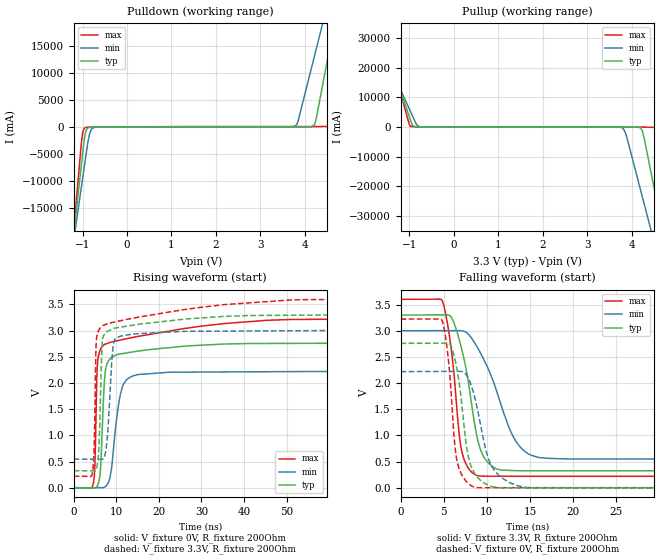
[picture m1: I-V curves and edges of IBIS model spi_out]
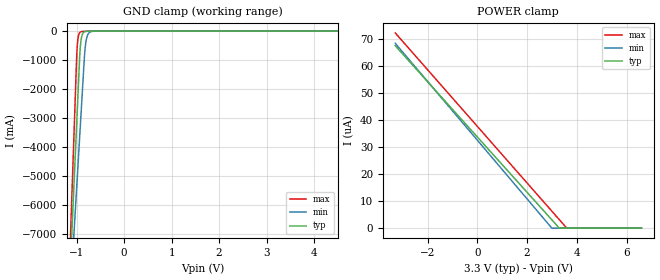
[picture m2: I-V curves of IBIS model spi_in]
|Texas Instruments Incorporated
| Part Name   Digital Voltage Range   Package-type   #pins
| DRV3245AQPHPRQ1   3 - 3.6 V   HTQFP   48
[IBIS Ver]   4.1
[File name]   drv3245_q1.ibs
[File Rev]   1.0
[Date]   06/05/2019
[Source]
| Texas Instruments Incorporated.
| 12500 TI Blvd
| Dallas, TX -75243
[Notes]   Revision History:
| Rev 1.0: 06/05/2019
| - Initial version of the model
| - Model generated from simulations in TISPICE/SPECTRE
| - C_comp although listed in numerical order of value are
|   obtained from varying PVT conditions. For PVT conditions for
|   each specific value refer the buffer description under
|   respective [Model]. IBIS model user is responsible for using
|   appropriate C_comp to simulate for Signal Integrity.
| - Warnings regarding combined Non-monotonicity of various models have been
|   reviewed and considered minor and can be ignored.
[Disclaimer]
| This model is designed as an aid for customers of Texas Instruments.
| TI and its licensors and suppliers make no warranties, either expressed
| or implied, with respect to this  model, including the warranties of
| merchantability or fitness for a particular purpose. The model is
| provided solely on an "as is" basis. The entire risk as to its quality
| and performance is with the customer.
| This model is subject to change without notice. Texas Instruments
| Incorporated is not responsible for updating this model.
[Copyright]
 (C) Copyright 2019 Texas Instruments Incorporated. All rights reserved.
|   DRV3245QPHPRQ1
[Component] DRV3245QPHPRQ1
[Manufacturer]   TI
[Package]
| variable   typ   min   max
R_pkg   0.05   0.04   0.06
L_pkg   1.0nH   0.8nH   1.2nH
C_pkg   0.2pF   0.16pF   0.24pF
| pin number (pin name) mapping to model name
[Pin]   signal_name   model_name   R_pin   L_pin   C_pin
1   EN   NC   NA   NA   NA
2   INHA   NC   NA   NA   NA
3   INLA   NC   NA   NA   NA
4   INHB   NC   NA   NA   NA
5   INLB   NC   NA   NA   NA
6   INHC   NC   NA   NA   NA
7   INLC   NC   NA   NA   NA
8   nFAULT   NC   NA   NA   NA
9   nSCS   spi_in   NA   NA   NA
10   SDI   spi_in   NA   NA   NA
11   SDO   spi_out   NA   NA   NA
12   SCLK   spi_in   NA   NA   NA
13   VDDIO   NC   NA   NA   NA
14   GND   GND   NA   NA   NA
15   AVDD   POWER   NA   NA   NA
16   SO1   NC   NA   NA   NA
17   SO2   NC   NA   NA   NA
18   SO3   NC   NA   NA   NA
19   SN3   NC   NA   NA   NA
20   SP3   NC   NA   NA   NA
21   SN2   NC   NA   NA   NA
22   SP2   NC   NA   NA   NA
23   SN1   NC   NA   NA   NA
24   SP1   NC   NA   NA   NA
25   GLC   NC   NA   NA   NA
26   SLC   NC   NA   NA   NA
27   SHC   NC   NA   NA   NA
28   GHC   NC   NA   NA   NA
29   GHB   NC   NA   NA   NA
30   SHB   NC   NA   NA   NA
31   SLB   NC   NA   NA   NA
32   GLB   NC   NA   NA   NA
33   GLA   NC   NA   NA   NA
34   SLA   NC   NA   NA   NA
35   SHA   NC   NA   NA   NA
36   GHA   NC   NA   NA   NA
37   VCP_LSD   NC   NA   NA   NA
38   VCPH   NC   NA   NA   NA
39   CP2H   NC   NA   NA   NA
40   CP2L   NC   NA   NA   NA
41   PVDD   NC   NA   NA   NA
42   CP1L   NC   NA   NA   NA
43   CP1H   NC   NA   NA   NA
44   VDRAIN   NC   NA   NA   NA
45   GND   NC   NA   NA   NA
46   DVDD   NC   NA   NA   NA
47   DRVOFF   NC   NA   NA   NA
48   VREF   NC   NA   NA   NA
| Models and submodels in the file (2): spi_out (Output), spi_in (Input)
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|   Model
[Model]   spi_out
Model_type   Output
Polarity   Non-Inverting
Vmeas = 1.65
Vref = 1.65
Cref = 15pF
Rref = 1000000
|   typ   min   max
C_comp   2.7pF   2.5pF   2.9pF
[Voltage Range]   3.3   3   3.6
[Temperature Range]   27   125   -40
[Pullup Reference]   3.3   3   3.6
[Pulldown Reference]   0   0   -0
[Power Clamp Reference]   3.3   3   3.6
[GND Clamp Reference]   0   0   0
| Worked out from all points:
|   slope of the pulldown table from 0 to 0.495 V, typ, clamps not added: 23.9 ohm
|   slope of the pullup table from 0 to 0.495 V, typ, clamps not added: 38.7 ohm
|   falling waveform, V_fixture 3.3V, R_fixture 200Ohm: 20-80 % time 1.94ns typ, 3.41ns min, 1.25ns max; typ from 3.3 V to 0.325 V
|   rising waveform, V_fixture 0V, R_fixture 200Ohm: 20-80 % time 978ps typ, 1.96ns min, 953ps max; typ from 0 V to 2.76 V
|   rising waveform, V_fixture 3.3V, R_fixture 200Ohm: 20-80 % time 662ps typ, 1.06ns min, 707ps max; typ from 0.325 V to 3.3 V
|   falling waveform, V_fixture 0V, R_fixture 200Ohm: 20-80 % time 1.31ns typ, 1.95ns min, 957ps max; typ from 2.76 V to 0 V
[Pulldown]
|   Voltage   I(typ)   I(min)   I(max)
-3.3V     -177.2A    -141.8A    -217.3A
-1.033V   -7.456A    -11.49A    -3.448A
-993.3mV  -4.492A    -9.214A    -914.7mA
-933.9mV  -1.068A    -5.8A      -112.1mA
-834.9mV  -62.44mA   -1.1A      -55.4mA
-716.1mV  -35.54mA   -62.31mA   -54.79mA
3.788V    36.46mA    202.9mA    61.09mA
3.848V    36.53mA    979.1mA    61.11mA
4.224V    470.4mA    13.29A     61.72mA
4.551V    14.09A     24A        129.5mA
4.61V     16.65A     25.95A     1.155A
6.6V      102.3A     91.21A     110.1A
[Pullup]
|   Voltage   I(typ)   I(min)   I(max)
-3.3V     102.3A     81.38A     126.5A
-1.013V   3.86A      6.372A     1.298A
-963.6mV  1.729A     4.748A     167.9mA
-844.8mV  50.39mA    901.1mA    42.5mA
-745.8mV  26.1mA     71.74mA    38.52mA
3.798V    -29.32mA   -419.2mA   -48.82mA
3.887V    -29.69mA   -3.169A    -48.9mA
4.234V    -1.069A    -23.04A    -50.85mA
4.283V    -3.752A    -25.89A    -52.93mA
4.551V    -23.76A    -41.25A    -182mA
4.63V     -29.69A    -45.81A    -3.197A
6.6V      -177.2A    -159.1A    -189A
[Ramp]
R_load = 200
|   typ   min   max
dV/dt_r   1.65554/9.78117e-10   1.33169/1.95563e-09   1.93285/9.39327e-10
dV/dt_f   1.78483/1.93755e-09   1.47239/3.40891e-09   2.02789/1.24785e-09
[Falling Waveform]
V_fixture = 3.3V
V_fixture_min = 3V
V_fixture_max = 3.6V
R_fixture = 200Ohm
C_fixture = 0F
|   Time   V(typ)   V(min)   V(max)
0s        3.3V       3V         3.6V
4.827ns   3.303V     3.001V     3.572V
5.882ns   3.255V     3.002V     2.636V
6.78ns    2.837V     3.002V     1.042V
7.109ns   2.626V     2.999V     685.5mV
8.867ns   967mV      2.693V     236.3mV
9.819ns   546.7mV    2.389V     223.2mV
13.73ns   328mV      804.3mV    221mV
19.54ns   326.2mV    550.7mV    220.4mV
1us       325.3mV    546mV      220.2mV
[Rising Waveform]
V_fixture = 0V
V_fixture_min = 0V
V_fixture_max = 0V
R_fixture = 200Ohm
C_fixture = 0F
|   Time   V(typ)   V(min)   V(max)
0s        -811.4pV   1.272nV    -234.2pV
4.596ns   -1.575mV   -99.85uV   76.49mV
5ns       -1.713mV   -108.6uV   482.5mV
5.558ns   35.75mV    93.74uV    2.336V
6.322ns   389.5mV    370.9uV    2.645V
6.969ns   1.648V     783.3uV    2.719V
8.13ns    2.417V     97.33mV    2.761V
12.69ns   2.576V     2.079V     2.849V
45.33ns   2.754V     2.214V     3.195V
1us       2.759V     2.219V     3.221V
[Rising Waveform]
V_fixture = 3.3V
V_fixture_min = 3V
V_fixture_max = 3.6V
R_fixture = 200Ohm
C_fixture = 0F
|   Time   V(typ)   V(min)   V(max)
0s        325.3mV    546mV      220.2mV
4.385ns   322.1mV    542.8mV    279mV
4.802ns   321.8mV    542.5mV    756.4mV
5.298ns   353.6mV    542.1mV    2.779V
5.972ns   867.9mV    541.6mV    3.016V
6.619ns   2.64V      541.1mV    3.085V
7.698ns   2.975V     798.3mV    3.124V
9.919ns   3.05V      2.859V     3.169V
50.77ns   3.292V     2.997V     3.583V
1us       3.3V       3V         3.6V
[Falling Waveform]
|Gnd
V_fixture = 0V
V_fixture_min = 0V
V_fixture_max = 0V
R_fixture = 200Ohm
C_fixture = 0F
|   Time   V(typ)   V(min)   V(max)
0s        2.759V     2.219V     3.221V
4.802ns   2.763V     2.223V     3.197V
5.504ns   2.761V     2.223V     2.502V
6.254ns   2.493V     2.224V     871mV
6.57ns    2.234V     2.224V     493.7mV
7.816ns   621.8mV    2.102V     89.25mV
8.98ns    190.3mV    1.446V     2.492mV
10.77ns   17.95mV    357.5mV    2.487mV
15.26ns   2.263mV    2.775mV    2.476mV
1us       -726.9pV   1.404nV    -192.1pV
|   Mode2
[Model]   spi_in
Model_type   Input
Vinl = 0.99
Vinh = 2.31
|   typ   min   max
C_comp   1.45pF   1.35pF   1.55pF
[Voltage Range]   3.3   3   3.6
[Temperature Range]   27   125   -40
[Power Clamp Reference]   3.3   3   3.6
[GND Clamp Reference]   0   0   0
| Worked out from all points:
|   GND clamp passes 1 mA (typ) near -0.65 V on its own axis
[GND Clamp]
|   Voltage   I(typ)   I(min)   I(max)
-3.3V     -87.91A    -69.25A    -109.9A
-1.251V   -12.5A     -12.41A    -12.86A
-1.112V   -7.4A      -8.564A    -6.292A
-993.3mV  -3.03A     -5.27A     -719.9mA
-963.6mV  -1.937A    -4.447A    -185.8mA
-933.9mV  -857.1mA   -3.623A    -53.88mA
-914.1mV  -417.1mA   -3.074A    -27.29mA
-874.5mV  -101.3mA   -1.977A    -11.77mA
-815.1mV  -15.06mA   -513.1mA   -7.465mA
-765.6mV  -5.154mA   -131.8mA   -5.933mA
-686.4mV  -1.851mA   -15.88mA   -3.079mA
6.6V      0A         0A         0A
[POWER Clamp]
|   Voltage   I(typ)   I(min)   I(max)
-3.3V     67.36uA    68.26uA    72.08uA
2.996V    3.074uA    12.54nA    6.281uA
3.293V    41.46nA    0A         3.178uA
3.61V     0A         0A         0A
6.6V      0A         0A         0A
